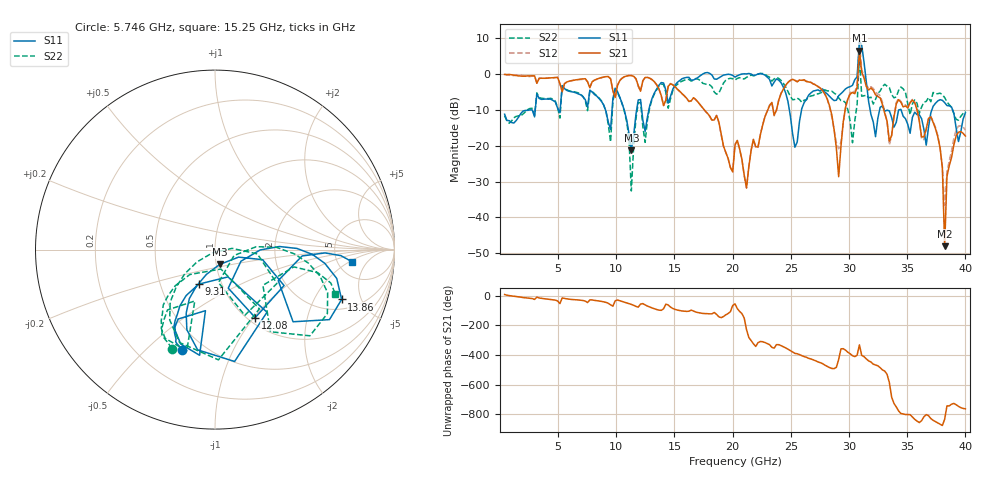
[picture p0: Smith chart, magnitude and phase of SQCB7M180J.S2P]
! Network Analyzer HP8722ES.07.66: Jul 25, 2000 Serial No. US39175408
! 27 Oct 2004  08:05:46
! Frequency  S11  S21  S12  S22
# HZ  S  DB R  50
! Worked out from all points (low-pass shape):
!   201 points, 400 MHz to 40 GHz, reference 50 ohm
!   highest |S21| = 6.52 dB at 30.89 GHz (marker M1); lowest = -48.0 dB at 38.22 GHz (marker M2)
!   |S21| within 3 dB of the highest: 30.83 GHz to 30.99 GHz (156.9 MHz wide, 0.508 % of centre)
!   lowest |S11| = -21.2 dB at 11.29 GHz (marker M3), VSWR 1.19, Z = 51.9 - j8.66 ohm
!   |S11| at or under -10 dB: start of sweep to 3.034 GHz; 33.02 GHz to 34.31 GHz (1.292 GHz wide, 3.84 % of centre); 34.47 GHz to 37.12 GHz (2.652 GHz wide, 7.41 % of centre)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
!   |S22| runs from -32.6 to 5.2 dB; largest |S21 - S12| = 0.97
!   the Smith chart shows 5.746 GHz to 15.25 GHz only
!   S11 on the Smith chart (normalised r, x): 5.746 GHz: 0.38, -0.66; 9.31 GHz: 0.78, -0.31; 12.08 GHz: 1.08, -1.02; 13.86 GHz: 2.59, -3.39; 15.25 GHz: 6.77, -2.16
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4e8  -11.23 -84.4  -0.14 7.9  -0.06 9.7  -11.65 -79.2
5.746e9  -4.59 -107.9  -2.24 -21.3  -2.25 -21.8  -4.42 -113.6
7.132e9  -6.32 -117.4  -1.38 -32.4  -1.50 -33.2  -6.30 -126.0
9.31e9  -13.45 -115.2  -0.73 -51.2  -0.75 -52.0  -14.11 -135.2
1.0498e10  -8.21 -114.4  -1.18 -38.6  -1.16 -39.5  -8.30 -130.5
1.129e10  -21.24 -72.6  -0.45 -58.7  -0.43 -59.3  -32.62 -128.6
1.2082e10  -7.13 -59.4  -4.81 -56.3  -4.75 -55.8  -7.91 -65.6
1.3666e10  -3.13 -13.3  -4.23 -97.3  -4.26 -97.3  -3.45 -21.0
1.3864e10  -2.40 -21.5  -6.06 -98.8  -6.07 -99.4  -2.85 -29.6
1.525e10  -2.34 -5.0  -4.28 -97.1  -4.26 -97.5  -2.92 -20.2
2.02e10  -0.87 -13.4  -19.86 -54.8  -19.57 -55.8  -1.71 -24.7
2.6932e10  -4.75 34.6  -2.81 -73.4  -2.77 -71.8  -6.01 -26.0
2.911e10  -6.06 -178.7  -28.65 -69.7  -20.85 -66.0  -6.67 -146.6
3.0496e10  -1.59 92.6  -5.49 -51.3  -5.03 -52.0  -13.08 97.4
3.0694e10  -0.81 87.5  -3.72 -41.7  -3.02 -43.3  -8.54 133.2
3.0892e10  9.12 118.8  6.52 28.2  9.34 15.8  5.18 -111.9
3.109e10  7.97 -43.3  0.51 -42.9  1.15 -46.8  -6.19 -74.0
3.1684e10  -7.69 -105.3  -4.49 -80.1  -4.02 -82.4  -6.66 -10.4
3.3466e10  -10.29 -137.7  -18.73 133.3  -19.82 127.8  -3.81 -102.2
3.703e10  -10.84 -131.4  -11.96 -109.6  -11.84 -111.4  -7.74 165.3
3.8218e10  -7.99 166.5  -48.02 -114.4  -36.66 70.3  -6.59 140.2
4e10  -10.81 -166.2  -17.31 -44.1  -15.67 -49.1  -10.28 166.2
